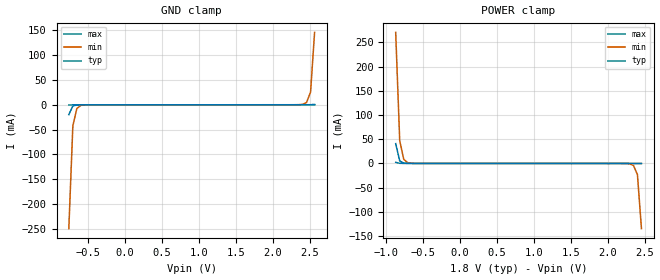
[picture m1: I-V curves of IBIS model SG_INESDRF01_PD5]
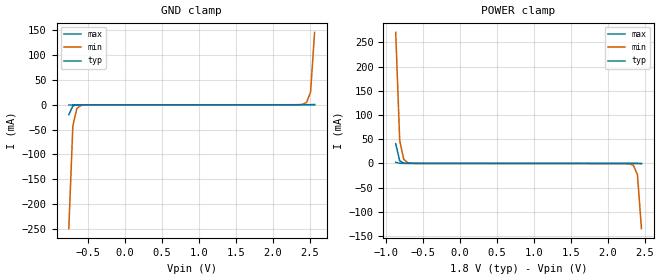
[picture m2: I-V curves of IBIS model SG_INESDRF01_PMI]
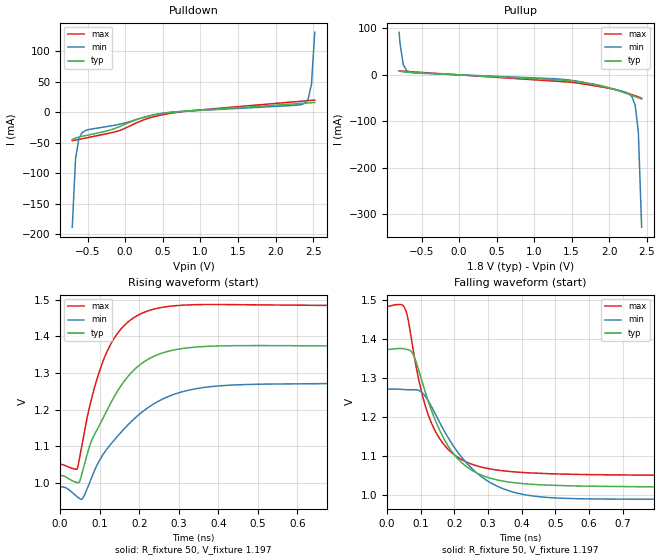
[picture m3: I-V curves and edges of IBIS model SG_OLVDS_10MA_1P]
|   This file is an IBIS representation of the   |
|   Integrated Device Technology Inc   |
|   IDT8P34S1204I   |
|   1:4 LVDS OUTPUT 1.8V FANOUT BUFFER   |
[IBIS Ver]   4.1
[File name]   8p34s1204i.ibs
[File Rev]   1.0
[Date]   6 Mar 2014
[Source]   Originated at Integrated Device Technology, Inc.
[Disclaimer]
IDT hereby grants the user of this IBIS model a non-exclusive,
nontransferable license to use this IBIS model under the following terms.
Before using this IBIS model, the user should read this license.
If the user does not accept these terms,  the IBIS model should be
returned to IDT within 30 days.
   The user is granted this license only to use the IBIS model and
is not granted rights to sell, load, rent, lease or license the IBIS
model in whole or in part, or in modified form to anyone other than
user. User may modify the IBIS model to suit its specific
applications but rights to derivative works and such modifications
shall belong to IDT.
   This IBIS model is provided on an "AS IS" basis and IDT makes
absolutely no warranty with respect to the information contained
herein. IDT DISCLAIMS AND CUSTOMER WAIVES ALL WARRANTIES, EXPRESS
OR IMPLIED, INCLUDING WARRANTIES OF MERCHANTABILITY OR FITNESS FOR
A PARTICULAR PURPOSE. The entire risk as to quality and performance
is with the Customer. ACCORDINGLY, IN NO EVENT SHALL THE COMPANY BE
LIABLE FOR ANY DAMAGES, WHETHER IN CONTRACT OR TORT,INCLUDING ANY
LOST PROFITS OR OTHER INCIDENTAL, CONSEQUENTIAL, EXEMPLARY, OR
PUNITIVE DAMAGES ARISING OUT OF THE USE OR APPLICATION OF THE IBIS
model provided in this package. Further, IDT reserves the right to
make changes without notice to any product herein to improve
reliability, function, or design. IDT does not convey any license
under patent rights or any other intellectual property rights,
including those of third parties.
   IDT is not obligated to provide maintenance or support
for the licensed IBIS model.
[Copyright] Copyright 2014 by Integrated Device Technology, Inc.
[Component]   IDT8P34S1204NLGI
[Manufacturer] Integrated Device Technology, Inc.
[Package]
|QFN 16
|lead + wire   typ   min   max
R_pkg   72.4655m   58.886m   86.045m
L_pkg   1.47175nH   1.11650nH   1.77850n
C_pkg   0.07747pF   0.07444pF   0.08050pF
[Pin] signal_name  model_name   R_pin   L_pin   C_pin
1   VEE   GND   86.045m   1.77850nH   0.08050pF
2   SEL   SG_INESDRF01_PD5   58.886m   1.11650nH   0.07444pF
3   PCLK1   SG_INESDRF01_PD5   58.886m   1.11650nH   0.07444pF
4   nPCLK1   SG_INESDRF01_PMI   86.045m   1.77850nH   0.08050pF
5   VCC   POWER   86.045m   1.77850nH   0.08050pF
6   PCLK0   SG_INESDRF01_PD5   58.886m   1.11650nH   0.07444pF
7   nPCLK0   SG_INESDRF01_PMI   58.886m   1.11650nH   0.07444pF
8   VREF   NC   86.045m   1.77850nH   0.08050pF
9   Q0   SG_OLVDS_10MA_1P   86.045m   1.77850nH   0.08050pF
10   nQ0   SG_OLVDS_10MA_1P   58.886m   1.11650nH   0.07444pF
11   Q1   SG_OLVDS_10MA_1P   58.886m   1.11650nH   0.07444pF
12   nQ1   SG_OLVDS_10MA_1P   86.045m   1.77850nH   0.08050pF
13   Q2   SG_OLVDS_10MA_1P   86.045m   1.77850nH   0.08050pF
14   nQ2   SG_OLVDS_10MA_1P   58.886m   1.11650nH   0.07444pF
15   Q3   SG_OLVDS_10MA_1P   58.886m   1.11650nH   0.07444pF
16   nQ3   SG_OLVDS_10MA_1P   86.045m   1.77850nH   0.08050pF
[Diff Pin]  inv_pin   vdiff   tdelay_typ   tdelay_min   tdelay_max
3   4   0.2   NA   NA   NA
6   7   0.2   NA   NA   NA
9   10   NA   0   0   0
11   12   NA   0   0   0
13   14   NA   0   0   0
15   16   NA   0   0   0
| Models and submodels in the file (3): SG_INESDRF01_PD5 (Input), SG_INESDRF01_PMI (Input), SG_OLVDS_10MA_1P (Output)
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[Model]   SG_INESDRF01_PD5
Model_type   Input
Polarity   Non-Inverting
Vinl = 0.5775V
Vinh = 1.2675V
|   typ   min   max
C_comp   2pF   1.5pF   2.5pF
|   typ   min   max
[Voltage range]   1.8V   1.65V   1.95V
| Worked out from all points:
|   GND clamp passes 1 mA (typ) near -0.67 V on its own axis
|   POWER clamp passes 1 mA (typ) near -0.77 V on its own axis
[GND_clamp]
|Voltage   I (typ)   I (min)   I (max)
|Note, modeling breaks down at 250mA and above.  This is well beyond the functional   |
|operating range of the device.  Should this scenario occur, catastrophic failure and   |
|possible damage to the device and/or board is of higher concern than the I-V curve   |
|behavior.  The IBIS checker will flag currents in excess of 10A with warnings.  Lines   |
|with currents in excess of 0.35 A have been commented out.  The points still remain|
|available to the user if the user desires to use them.   |
|-1.80000e+00   -6.34663e+07   -4.98790e+07   -8.64483e+07
|-1.74545e+00   -5.65132e+07   -4.40907e+07   -7.75568e+07
|-1.69091e+00   -4.95601e+07   -3.83025e+07   -6.86652e+07
|-1.63636e+00   -4.26070e+07   -3.25142e+07   -5.97737e+07
|-1.58182e+00   -3.56539e+07   -2.67259e+07   -5.08821e+07
|-1.52727e+00   -2.87008e+07   -2.09377e+07   -4.19905e+07
|-1.47273e+00   -2.17477e+07   -1.51494e+07   -3.30990e+07
|-1.41818e+00   -1.47946e+07   -9.36113e+06   -2.42074e+07
|-1.36364e+00   -7.84151e+06   -3.89439e+06   -1.53159e+07
|-1.30909e+00   -2.62924e+06   -1.76457e+06   -6.42430e+06
|-1.25455e+00   -1.12653e+06   -8.19749e+05   -1.78119e+06
|-1.20000e+00   -2.49225e+05   -1.82061e+05   -4.56857e+05
|-1.14545e+00   -2.98386e+04   -3.11065e+04   -3.04223e+04
|-1.09091e+00   -3.58223e+03   -5.32383e+03   -2.02551e+03
|-1.03636e+00   -4.36536e+02   -9.17799e+02   -1.40352e+02
|-9.81818e-01   -5.64958e+01   -1.62416e+02   -1.19791e+01
|-9.27273e-01   -8.87847e+00   -3.09259e+01   -1.11285e+00
|-8.72727e-01   -1.39141e+00   -6.95910e+00   -7.37007e-02
|-8.18182e-01   -1.66516e-01   -1.46448e+00   -4.89952e-03
-763.6mV  -19.94mA   -250.1mA   -343uA
-709.1mV  -2.398mA   -42.72mA   -39.99uA
-654.5mV  -298.3uA   -7.304mA   -18.59uA
-600mV    -46.04uA   -1.255mA   -15.84uA
-490.9mV  -10.22uA   -43.56uA   -12.88uA
2.4V      48.77uA    848.8uA    62.97uA
2.455V    58.45uA    4.57mA     64.4uA
2.509V    130.8uA    25.48mA    65.84uA
2.564V    707.2uA    146.1mA    67.42uA
| 2.61818e+00   5.17747e-03   8.50177e-01   7.10820e-05
| 2.67273e+00   4.07785e-02   4.96920e+00   1.05333e-04
| 2.72727e+00   3.34701e-01   2.58351e+01   5.26598e-04
| 2.78182e+00   2.78621e+00   1.39432e+02   5.44315e-03
| 2.83636e+00   2.10020e+01   7.96021e+02   7.42575e-02
| 2.89091e+00   1.58647e+02   4.63214e+03   1.10491e+00
| 2.94545e+00   1.29328e+03   2.70862e+04   1.54370e+01
| 3.00000e+00   1.07595e+04   1.58559e+05   2.04192e+02
| 3.05455e+00   8.98499e+04   9.28397e+05   3.01684e+03
| 3.10909e+00   7.50771e+05   4.70872e+06   4.54605e+04
| 3.16364e+00   5.12124e+06   9.79622e+06   6.86489e+05
| 3.21818e+00   1.12326e+07   1.48837e+07   6.56736e+06
| 3.27273e+00   1.73439e+07   1.99712e+07   1.43824e+07
| 3.32727e+00   2.34552e+07   2.50587e+07   2.21975e+07
| 3.38182e+00   2.95665e+07   3.01462e+07   3.00126e+07
| 3.43636e+00   3.56778e+07   3.52337e+07   3.78277e+07
| 3.49091e+00   4.17891e+07   4.03212e+07   4.56428e+07
| 3.54545e+00   4.79004e+07   4.54087e+07   5.34579e+07
| 3.60000e+00   5.40117e+07   5.04962e+07   6.12730e+07
[Power_clamp]
|Voltage   I (typ)   I (min)   I (max)
|Note, modeling breaks down at 250mA and above.  This is well beyond the functional   |
|operating range of the device.  Should this scenario occur, catastrophic failure and   |
|possible damage to the device and/or board is of higher concern than the I-V curve   |
|behavior.  The IBIS checker will flag currents in excess of 10A with warnings.  Lines   |
|with currents in excess of 0.35 A have been commented out.  The points still remain|
|available to the user if the user desires to use them.   |
|-1.80000e+00   5.40117e+07   4.21018e+07   7.41679e+07
|-1.74545e+00   4.79004e+07   3.70143e+07   6.63528e+07
|-1.69091e+00   4.17891e+07   3.19268e+07   5.85377e+07
|-1.63636e+00   3.56778e+07   2.68393e+07   5.07226e+07
|-1.58182e+00   2.95665e+07   2.17518e+07   4.29075e+07
|-1.52727e+00   2.34552e+07   1.66643e+07   3.50924e+07
|-1.47273e+00   1.73439e+07   1.15768e+07   2.72773e+07
|-1.41818e+00   1.12326e+07   6.48935e+06   1.94623e+07
|-1.36364e+00   5.12124e+06   1.72338e+06   1.16472e+07
|-1.30909e+00   7.50771e+05   2.94324e+05   3.83208e+06
|-1.25455e+00   8.98499e+04   5.02724e+04   2.65438e+05
|-1.20000e+00   1.07595e+04   8.59233e+03   1.75828e+04
|-1.14545e+00   1.29328e+03   1.47285e+03   1.17022e+03
|-1.09091e+00   1.58647e+02   2.55533e+02   8.10441e+01
|-1.03636e+00   2.10025e+01   4.61765e+01   6.39596e+00
|-9.81818e-01   2.78656e+00   8.95678e+00   4.28158e-01
|-9.27273e-01   3.34942e-01   1.57738e+00   2.92320e-02
-872.7mV  40.91mA    270.8mA    2.305mA
-818.2mV  5.227mA    47.07mA    261.6uA
-763.6mV  730.3uA    8.405mA    83.44uA
-709.1mV  151.2uA    1.565mA    69.12uA
-600mV    68.27uA    112.2uA    65.33uA
2.291V    -14.21uA   -687.8uA   -10.52uA
2.345V    -19.34uA   -3.948mA   -11.95uA
2.4V      -50.92uA   -23.03mA   -13.38uA
2.455V    -303.6uA   -134.8mA   -14.83uA
| 2.50909e+00   -2.40403e-03   -7.88939e-01   -1.64856e-05
| 2.56364e+00   -1.99454e-02   -4.23150e+00   -2.13358e-05
| 2.61818e+00   -1.66523e-01   -1.79578e+01   -7.44084e-05
| 2.67273e+00   -1.39142e+00   -8.97511e+01   -8.55828e-04
| 2.72727e+00   -8.87848e+00   -4.98310e+02   -1.26382e-02
| 2.78182e+00   -5.64958e+01   -2.87349e+03   -1.90577e-01
| 2.83636e+00   -4.36536e+02   -1.67644e+04   -2.82774e+00
| 2.89091e+00   -3.58223e+03   -9.80861e+04   -2.70677e+01
| 2.94545e+00   -2.98386e+04   -5.51294e+05   -3.53671e+02
| 3.00000e+00   -2.49225e+05   -1.38353e+06   -5.22068e+03
| 3.05455e+00   -1.12653e+06   -2.85414e+06   -7.86550e+04
| 3.10909e+00   -2.62924e+06   -7.33524e+06   -8.61501e+05
| 3.16364e+00   -7.84151e+06   -1.31235e+07   -2.57900e+06
| 3.21818e+00   -1.47946e+07   -1.89118e+07   -9.53635e+06
| 3.27273e+00   -2.17477e+07   -2.47000e+07   -1.84279e+07
| 3.32727e+00   -2.87008e+07   -3.04883e+07   -2.73195e+07
| 3.38182e+00   -3.56539e+07   -3.62766e+07   -3.62110e+07
| 3.43636e+00   -4.26070e+07   -4.20648e+07   -4.51026e+07
| 3.49091e+00   -4.95601e+07   -4.78531e+07   -5.39942e+07
| 3.54545e+00   -5.65132e+07   -5.36414e+07   -6.28857e+07
| 3.60000e+00   -6.34663e+07   -5.94296e+07   -7.17773e+07
[Model]   SG_INESDRF01_PMI
Model_type   Input
Polarity   Non-Inverting
Vinl = 0.5775V
Vinh = 1.2675V
|   typ   min   max
C_comp   2pF   1.5pF   2.5pF
|   typ   min   max
[Voltage range]   1.8V   1.65V   1.95V
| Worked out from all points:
|   GND clamp passes 1 mA (typ) near -0.67 V on its own axis
|   POWER clamp passes 1 mA (typ) near -0.77 V on its own axis
[GND_clamp]
|Voltage   I (typ)   I (min)   I (max)
|Note, modeling breaks down at 250mA and above.  This is well beyond the functional   |
|operating range of the device.  Should this scenario occur, catastrophic failure and   |
|possible damage to the device and/or board is of higher concern than the I-V curve   |
|behavior.  The IBIS checker will flag currents in excess of 10A with warnings.  Lines   |
|with currents in excess of 0.35 A have been commented out.  The points still remain|
|available to the user if the user desires to use them.   |
|-1.80000e+00   -6.34663e+07   -4.98790e+07   -8.64483e+07
|-1.74545e+00   -5.65132e+07   -4.40907e+07   -7.75568e+07
|-1.69091e+00   -4.95601e+07   -3.83025e+07   -6.86652e+07
|-1.63636e+00   -4.26070e+07   -3.25142e+07   -5.97737e+07
|-1.58182e+00   -3.56539e+07   -2.67259e+07   -5.08821e+07
|-1.52727e+00   -2.87008e+07   -2.09377e+07   -4.19905e+07
|-1.47273e+00   -2.17477e+07   -1.51494e+07   -3.30990e+07
|-1.41818e+00   -1.47946e+07   -9.36113e+06   -2.42074e+07
|-1.36364e+00   -7.84151e+06   -3.89439e+06   -1.53159e+07
|-1.30909e+00   -2.62924e+06   -1.76457e+06   -6.42430e+06
|-1.25455e+00   -1.12653e+06   -8.19749e+05   -1.78119e+06
|-1.20000e+00   -2.49225e+05   -1.82061e+05   -4.56857e+05
|-1.14545e+00   -2.98386e+04   -3.11065e+04   -3.04223e+04
|-1.09091e+00   -3.58223e+03   -5.32383e+03   -2.02551e+03
|-1.03636e+00   -4.36536e+02   -9.17799e+02   -1.40352e+02
|-9.81818e-01   -5.64958e+01   -1.62416e+02   -1.19791e+01
|-9.27273e-01   -8.87853e+00   -3.09260e+01   -1.11292e+00
|-8.72727e-01   -1.39146e+00   -6.95914e+00   -7.37732e-02
|-8.18182e-01   -1.66568e-01   -1.46452e+00   -4.97058e-03
-763.6mV  -19.99mA   -250.1mA   -412.6uA
-709.1mV  -2.448mA   -42.76mA   -108.2uA
-654.5mV  -347uA     -7.339mA   -85.35uA
-600mV    -93.63uA   -1.289mA   -81.17uA
-490.9mV  -55.65uA   -75.99uA   -75.35uA
2.4V      60.67uA    859uA      76.35uA
2.455V    71.43uA    4.581mA    79.21uA
2.509V    144.8uA    25.49mA    82.09uA
2.564V    722.4uA    146.2mA    85.1uA
| 2.61818e+00   5.19369e-03   8.50190e-01   9.01874e-05
| 2.67273e+00   4.07959e-02   4.96921e+00   1.25870e-04
| 2.72727e+00   3.34719e-01   2.58352e+01   5.48566e-04
| 2.78182e+00   2.78623e+00   1.39432e+02   5.46655e-03
| 2.83636e+00   2.10020e+01   7.96021e+02   7.42824e-02
| 2.89091e+00   1.58647e+02   4.63214e+03   1.10493e+00
| 2.94545e+00   1.29328e+03   2.70862e+04   1.54370e+01
| 3.00000e+00   1.07595e+04   1.58559e+05   2.04192e+02
| 3.05455e+00   8.98499e+04   9.28397e+05   3.01684e+03
| 3.10909e+00   7.50771e+05   4.70872e+06   4.54605e+04
| 3.16364e+00   5.12124e+06   9.79622e+06   6.86489e+05
| 3.21818e+00   1.12326e+07   1.48837e+07   6.56736e+06
| 3.27273e+00   1.73439e+07   1.99712e+07   1.43824e+07
| 3.32727e+00   2.34552e+07   2.50587e+07   2.21975e+07
| 3.38182e+00   2.95665e+07   3.01462e+07   3.00126e+07
| 3.43636e+00   3.56778e+07   3.52337e+07   3.78277e+07
| 3.49091e+00   4.17891e+07   4.03212e+07   4.56428e+07
| 3.54545e+00   4.79004e+07   4.54087e+07   5.34579e+07
| 3.60000e+00   5.40117e+07   5.04962e+07   6.12730e+07
[Power_clamp]
|Voltage   I (typ)   I (min)   I (max)
|Note, modeling breaks down at 250mA and above.  This is well beyond the functional   |
|operating range of the device.  Should this scenario occur, catastrophic failure and   |
|possible damage to the device and/or board is of higher concern than the I-V curve   |
|behavior.  The IBIS checker will flag currents in excess of 10A with warnings.  Lines   |
|with currents in excess of 0.35 A have been commented out.  The points still remain|
|available to the user if the user desires to use them.   |
|-1.80000e+00   5.40117e+07   4.21018e+07   7.41679e+07
|-1.74545e+00   4.79004e+07   3.70143e+07   6.63528e+07
|-1.69091e+00   4.17891e+07   3.19268e+07   5.85377e+07
|-1.63636e+00   3.56778e+07   2.68393e+07   5.07226e+07
|-1.58182e+00   2.95665e+07   2.17518e+07   4.29075e+07
|-1.52727e+00   2.34552e+07   1.66643e+07   3.50924e+07
|-1.47273e+00   1.73439e+07   1.15768e+07   2.72773e+07
|-1.41818e+00   1.12326e+07   6.48935e+06   1.94623e+07
|-1.36364e+00   5.12124e+06   1.72338e+06   1.16472e+07
|-1.30909e+00   7.50771e+05   2.94324e+05   3.83208e+06
|-1.25455e+00   8.98499e+04   5.02724e+04   2.65438e+05
|-1.20000e+00   1.07595e+04   8.59233e+03   1.75828e+04
|-1.14545e+00   1.29328e+03   1.47285e+03   1.17022e+03
|-1.09091e+00   1.58647e+02   2.55533e+02   8.10441e+01
|-1.03636e+00   2.10025e+01   4.61765e+01   6.39599e+00
|-9.81818e-01   2.78659e+00   8.95681e+00   4.28184e-01
|-9.27273e-01   3.34968e-01   1.57740e+00   2.92564e-02
-872.7mV  40.93mA    270.8mA    2.328mA
-818.2mV  5.25mA     47.09mA    283uA
-763.6mV  751.6uA    8.427mA    103.5uA
-709.1mV  171uA      1.586mA    87.72uA
-600mV    85.05uA    129.6uA    81.08uA
2.291V    -78.26uA   -754uA     -70.63uA
2.345V    -84.91uA   -4.015mA   -73.49uA
2.4V      -118uA     -23.1mA    -76.35uA
2.455V    -372.2uA   -134.8mA   -79.23uA
| 2.50909e+00   -2.47418e-03   -7.89012e-01   -8.23171e-05
| 2.56364e+00   -2.00171e-02   -4.23158e+00   -8.85984e-05
| 2.61818e+00   -1.66596e-01   -1.79579e+01   -1.43102e-04
| 2.67273e+00   -1.39149e+00   -8.97512e+01   -9.25953e-04
| 2.72727e+00   -8.87856e+00   -4.98310e+02   -1.27097e-02
| 2.78182e+00   -5.64959e+01   -2.87349e+03   -1.90650e-01
| 2.83636e+00   -4.36536e+02   -1.67644e+04   -2.82782e+00
| 2.89091e+00   -3.58223e+03   -9.80861e+04   -2.70678e+01
| 2.94545e+00   -2.98386e+04   -5.51294e+05   -3.53671e+02
| 3.00000e+00   -2.49225e+05   -1.38353e+06   -5.22068e+03
| 3.05455e+00   -1.12653e+06   -2.85414e+06   -7.86550e+04
| 3.10909e+00   -2.62924e+06   -7.33524e+06   -8.61501e+05
| 3.16364e+00   -7.84151e+06   -1.31235e+07   -2.57900e+06
| 3.21818e+00   -1.47946e+07   -1.89118e+07   -9.53635e+06
| 3.27273e+00   -2.17477e+07   -2.47000e+07   -1.84279e+07
| 3.32727e+00   -2.87008e+07   -3.04883e+07   -2.73195e+07
| 3.38182e+00   -3.56539e+07   -3.62766e+07   -3.62110e+07
| 3.43636e+00   -4.26070e+07   -4.20648e+07   -4.51026e+07
| 3.49091e+00   -4.95601e+07   -4.78531e+07   -5.39942e+07
| 3.54545e+00   -5.65132e+07   -5.36414e+07   -6.28857e+07
| 3.60000e+00   -6.34663e+07   -5.94296e+07   -7.17773e+07
[Model]   SG_OLVDS_10MA_1P
Model_type   Output
Polarity   Non-Inverting
|   typ   min   max
C_comp   2pF   1.5pF   2.5pF
Vmeas = 1.222V
Rref = 50
Cref = 0
Vref = 1.222V
|   typ   min   max
[Voltage range]   1.8V   1.71V   1.89V
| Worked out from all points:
|   slope of the pulldown table from 0 to 0.27 V, typ, clamps not added: 22.6 ohm
|   slope of the pullup table from 0 to 0.27 V, typ, clamps not added: 121 ohm
|   rising waveform, R_fixture 50, V_fixture 1.197: 20-80 % time 110ps typ, 144ps min, 76.8ps max; typ from 1.02 V to 1.37 V
|   falling waveform, R_fixture 50, V_fixture 1.197: 20-80 % time 113ps typ, 144ps min, 89.3ps max; typ from 1.37 V to 1.02 V
[Pulldown]
|Voltage   I (typ)   I (min)   I (max)
|Note, modeling breaks down at 250mA and above.  This is well beyond the functional   |
|operating range of the device.  Should this scenario occur, catastrophic failure and   |
|possible damage to the device and/or board is of higher concern than the I-V curve   |
|behavior.  The IBIS checker will flag currents in excess of 10A with warnings.  Lines   |
|with currents in excess of 0.35 A have been commented out.  The points still remain|
|available to the user if the user desires to use them.   |
|-1.60000e+00   -3.79716e+07   -2.40942e+07   -5.38460e+07
|-1.40000e+00   -1.24769e+07   -5.00966e+06   -2.12436e+07
|-1.20000e+00   -2.49225e+05   -1.59031e+05   -4.56857e+05
|-1.00000e+00   -1.10440e+02   -4.77352e+02   -2.60627e+01
|-8.00000e-01   -1.27680e-01   -2.62740e+00   -5.12242e-02
|-7.90000e-01   -1.00915e-01   -1.98783e+00   -5.02020e-02
|-7.46437e-01   -5.43043e-02   -5.84371e-01   -4.80620e-02
-702.9mV  -44.85mA   -188.5mA   -46.86mA
-659.3mV  -42.21mA   -76mA      -45.76mA
-615.7mV  -40.81mA   -43.42mA   -44.67mA
-572.2mV  -39.64mA   -33.55mA   -43.58mA
-485.1mV  -37.37mA   -28.59mA   -41.37mA
-92.99mV  -24.55mA   -20.26mA   -30.83mA
212mV     -9.797mA   -9.696mA   -14.3mA
473.3mV   -2.449mA   -2.179mA   -4.859mA
2.39V     14.78mA    14.66mA    18.49mA
2.434V    15.14mA    21.64mA    18.95mA
2.477V    15.52mA    45.77mA    19.41mA
2.521V    15.96mA    130.9mA    19.87mA
| 2.56437e+00   1.68027e-02   4.33326e-01   2.03304e-02
| 2.60793e+00   1.97745e-02   1.50912e+00   2.07921e-02
| 2.65149e+00   3.43765e-02   5.33262e+00   2.12595e-02
| 2.69506e+00   1.12362e-01   1.73951e+01   2.17774e-02
| 2.73862e+00   5.35786e-01   5.70854e+01   2.27369e-02
| 2.78218e+00   2.84183e+00   1.95128e+02   2.75581e-02
| 2.82575e+00   1.43687e+01   6.83295e+02   6.61440e-02
| 2.86931e+00   7.02916e+01   2.41787e+03   3.99957e-01
| 2.91287e+00   3.67522e+02   8.58956e+03   3.31512e+00
| 2.95644e+00   1.97986e+03   3.05569e+04   2.56004e+01
| 3.00000e+00   1.07595e+04   1.08755e+05   2.04214e+02
| 3.01000e+00   1.58754e+04   1.45554e+05   3.33215e+02
| 3.12800e+00   1.56726e+06   4.18761e+06   1.16501e+05
| 3.24600e+00   1.43493e+07   1.40879e+07   1.05531e+07
| 3.36400e+00   2.75701e+07   2.39881e+07   2.74597e+07
| 3.48200e+00   4.07909e+07   3.38883e+07   4.43663e+07
| 3.60000e+00   5.40117e+07   4.37886e+07   6.12730e+07
[Pullup]
|Voltage   I (typ)   I (min)   I (max)
|Note, modeling breaks down at 250mA and above.  This is well beyond the functional   |
|operating range of the device.  Should this scenario occur, catastrophic failure and   |
|possible damage to the device and/or board is of higher concern than the I-V curve   |
|behavior.  The IBIS checker will flag currents in excess of 10A with warnings.  Lines   |
|with currents in excess of 0.35 A have been commented out.  The points still remain|
|available to the user if the user desires to use them.   |
|-1.60000e+00   3.16036e+07   1.94575e+07   4.55125e+07
|-1.40000e+00   9.19545e+06   2.68427e+06   1.68572e+07
|-1.20000e+00   1.07595e+04   7.90005e+03   1.75828e+04
|-1.00000e+00   5.64373e+00   2.60147e+01   1.06471e+00
-800mV    8.947mA    91.53mA    8.519mA
-790mV    8.106mA    69.69mA    8.394mA
-746.4mV  6.448mA    23.12mA    7.906mA
-702.9mV  5.851mA    9.833mA    7.442mA
-659.3mV  5.449mA    5.895mA    6.981mA
1.388V    -11.45mA   -9.682mA   -14.67mA
1.867V    -22.3mA    -23.05mA   -25.1mA
2.259V    -41.62mA   -40.22mA   -40.07mA
2.303V    -44.13mA   -46.45mA   -42.46mA
2.347V    -46.65mA   -64.2mA    -44.91mA
2.39V     -49.2mA    -122.9mA   -47.41mA
2.434V    -51.83mA   -327.5mA   -49.93mA
| 2.47724e+00   -5.49299e-02   -1.05110e+00   -5.24648e-02
| 2.52080e+00   -6.05302e-02   -3.46712e+00   -5.50106e-02
| 2.56437e+00   -7.97915e-02   -9.62257e+00   -5.75624e-02
| 2.60793e+00   -1.73529e-01   -2.82789e+01   -6.01402e-02
| 2.65149e+00   -6.73190e-01   -9.14306e+01   -6.29439e-02
| 2.69506e+00   -3.27216e+00   -3.11438e+02   -6.77359e-02
| 2.73862e+00   -1.28238e+01   -1.08814e+03   -8.99327e-02
| 2.78218e+00   -5.73228e+01   -3.84660e+03   -2.64332e-01
| 2.82575e+00   -2.91244e+02   -1.36600e+04   -1.76955e+00
| 2.86931e+00   -1.55165e+03   -4.85881e+04   -1.08837e+01
| 2.91287e+00   -8.40568e+03   -1.72922e+05   -7.39726e+01
| 2.95644e+00   -4.57446e+04   -5.81258e+05   -6.05587e+02
| 3.00000e+00   -2.49225e+05   -1.16290e+06   -5.22076e+03
| 3.01000e+00   -3.67806e+05   -1.31527e+06   -8.57981e+03
| 3.12800e+00   -3.73756e+06   -6.72102e+06   -1.30572e+06
| 3.24600e+00   -1.83407e+07   -1.79850e+07   -1.40710e+07
| 3.36400e+00   -3.33826e+07   -2.92489e+07   -3.33065e+07
| 3.48200e+00   -4.84244e+07   -4.05128e+07   -5.25419e+07
| 3.60000e+00   -6.34663e+07   -5.17768e+07   -7.17773e+07
[Ramp]
|   typ   min   max
dV/dt_r   0.224/0.111n   0.189/0.145n   0.269/0.078n
dV/dt_f   0.212/0.112n   0.168/0.143n   0.261/0.089n
R_load =   50.0000
[Rising Waveform]
R_fixture = 50
V_fixture   =1.197  |Vcc_typ
V_fixture_min=1.131  |Vcc_min
V_fixture_max=1.267  |Vcc_max
C_fixture = 0.0p
| Time   typ   min   max
0s        1.021V     989.9mV    1.051V
43.04ps   1.002V     963mV      1.039V
57.06ps   1.033V     959.1mV    1.115V
78.08ps   1.112V     1.012V     1.224V
115.1ps   1.191V     1.088V     1.35V
157.2ps   1.27V      1.142V     1.424V
212.2ps   1.331V     1.198V     1.465V
291.3ps   1.363V     1.243V     1.483V
395.4ps   1.373V     1.264V     1.486V
1ns       1.373V     1.272V     1.483V
[Falling Waveform]
R_fixture = 50
V_fixture   =1.197  |Vcc_typ
V_fixture_min=1.131  |Vcc_min
V_fixture_max=1.267  |Vcc_max
C_fixture = 0.0p
| Time   typ   min   max
0s        1.372V     1.272V     1.482V
50.05ps   1.375V     1.271V     1.482V
75.08ps   1.364V     1.27V      1.385V
102.1ps   1.297V     1.264V     1.266V
133.1ps   1.215V     1.226V     1.183V
179.2ps   1.13V      1.151V     1.12V
227.2ps   1.08V      1.092V     1.089V
312.3ps   1.043V     1.03V      1.067V
422.4ps   1.029V     1V         1.058V
1ns       1.021V     990.2mV    1.051V
